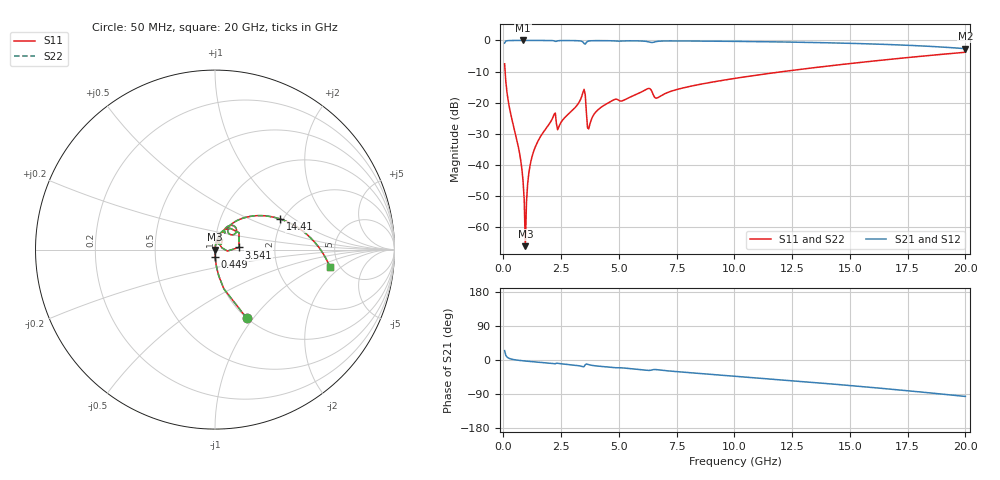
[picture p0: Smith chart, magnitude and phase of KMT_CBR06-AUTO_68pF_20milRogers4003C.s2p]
! Data measured by Modelithics Inc. support@modelithics.com 813-866-6335
! KEMET CBR06-AUTO 68pF, Pad Width= 0.851mm, Pad Length= 0.64mm, Pad Gap= 0.62mm, 20mil Rogers 4003C substrate Data, January 2022
# hz S ma R 50
! 2 Port Network Data from SP1.SP block
! freq  magS11  angS11  magS21  angS21  magS12  angS12  magS22  angS22
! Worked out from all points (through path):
!   401 points, 50 MHz to 20 GHz, reference 50 ohm
!   highest |S21| = 0.00 dB at 848 MHz (marker M1); lowest = -2.6 dB at 20 GHz (marker M2)
!   group delay of S21, straight-line fit = 13.4 ps
!   lowest |S11| = -66.1 dB at 947.8 MHz (marker M3), VSWR 1.00, Z = 50 - j0.00739 ohm
!   |S11| at or under -10 dB: 72.8 MHz to 12.1 GHz (12.03 GHz wide, 198 % of centre)
!   |S22| runs from -66.1 to -3.8 dB; largest |S21 - S12| = 0
!   S11 on the Smith chart (normalised r, x): 50 MHz: 1.00, -0.93; 449 MHz: 1.00, -0.08; 3.541 GHz: 1.31, +0.03; 14.41 GHz: 1.94, +0.79; 20 GHz: 4.19, -1.36
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5e7  0.4214 -65.2  0.9065 24.8  0.9065 24.8  0.4214 -65.2
4.49e8  0.04036 -88.5  0.9988 1.0  0.9988 1.0  0.04036 -88.5
7.4825e8  0.01188 -89.4  0.9995 -1.5  0.9995 -1.5  0.01188 -89.4
8.48e8  0.005606 -87.3  0.9995 -2.1  0.9995 -2.1  0.005606 -87.3
9.4775e8  0.000497 -8.5  0.9995 -2.7  0.9995 -2.7  0.000497 -8.5
1.0475e9  0.004991 80.7  0.9994 -3.3  0.9994 -3.3  0.004991 80.7
1.097375e9  0.007343 82.2  0.9994 -3.6  0.9994 -3.6  0.007343 82.2
1.197125e9  0.01183 83.2  0.9993 -4.1  0.9993 -4.1  0.01183 83.2
1.54625e9  0.02626 82.5  0.9989 -5.9  0.9989 -5.9  0.02626 82.5
2.14475e9  0.05847 74.6  0.9922 -9.5  0.9922 -9.5  0.05847 74.6
2.444e9  0.04481 74.4  0.9942 -9.5  0.9942 -9.5  0.04481 74.4
3.391625e9  0.1272 62.5  0.9687 -16.9  0.9687 -16.9  0.1272 62.5
3.54125e9  0.1336 5.2  0.8718 -12.4  0.8718 -12.4  0.1336 5.2
3.74075e9  0.04491 59.0  0.9852 -13.1  0.9852 -13.1  0.04491 59.0
4.788125e9  0.1117 65.1  0.9841 -20.1  0.9841 -20.1  0.1117 65.1
6.2345e9  0.1675 53.2  0.9582 -27.3  0.9582 -27.3  0.1675 53.2
6.73325e9  0.1235 54.7  0.9727 -26.2  0.9727 -26.2  0.1235 54.7
1.0025e10  0.2461 46.7  0.9661 -42.7  0.9661 -42.7  0.2461 46.7
1.336662e10  0.3621 30.5  0.9277 -58.9  0.9277 -58.9  0.3621 30.5
1.4414e10  0.4021 25.0  0.9103 -64.3  0.9103 -64.3  0.4021 25.0
1.670825e10  0.4964 12.4  0.8593 -76.7  0.8593 -76.7  0.4964 12.4
2e10  0.6463 -8.4  0.7373 -96.2  0.7373 -96.2  0.6463 -8.4
